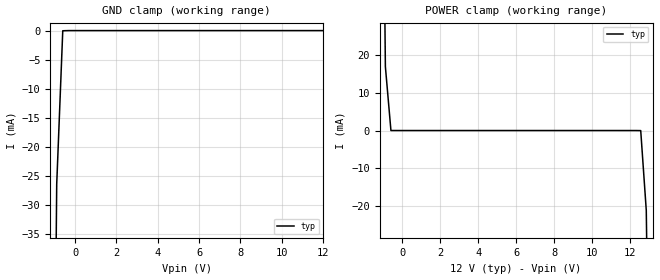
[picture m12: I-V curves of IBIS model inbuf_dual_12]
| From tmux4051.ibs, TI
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| inbuf_dual_12
[Model]   inbuf_dual_12
Model_type   Input
Vinl = 0.8
Vinh = 1.35
|   typ   min   max
C_comp   1.598234e-12   NA   NA
[Voltage Range]   12   NA   NA
[Temperature Range]   27   NA   NA
[Power Clamp Reference]   12   NA   NA
[GND Clamp Reference]   0   NA   NA
[GND Clamp]
|   Voltage   I(typ)   I(min)   I(max)
-17V      -11.08A    NA         NA
-1.182V   -139.8mA   NA         NA
-888.9mV  -26.42mA   NA         NA
-596mV    -30.87uA   NA         NA
12V       465nA      NA         NA
[POWER Clamp]
|   Voltage   I(typ)   I(min)   I(max)
-5V       3.679A     NA         NA
-1.192V   156.9mA    NA         NA
-899mV    16.91mA    NA         NA
-606.1mV  2.001uA    NA         NA
12.58V    -17.72uA   NA         NA
12.87V    -21.13mA   NA         NA
13.16V    -130.5mA   NA         NA
24V       -7.582A    NA         NA
